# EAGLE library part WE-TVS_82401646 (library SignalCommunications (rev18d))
TVS Diode Super Speed Series Characteristics Operating temperature: –55 ºC to +85 °C for 824 014 x; –40 ºC to +85 °C for 824 016 46 Low clamping voltage Very low capacitance Rail to Rail protection Epoxy flame resistant UL94 V-0 RoHS, REACH and free of halogens Applications Super Speed data lines HDMI 1.3/1.4, DVI DisplayPort USB 3.0 SuperSpeed SATA GBit LAN ESD protection in accordance with EN 61000-4-2 – 8 kV contact discharge – 15 kV air discharge Updated by Dan Xu 2014-07-11 2014 (C) Wurth Elektronik
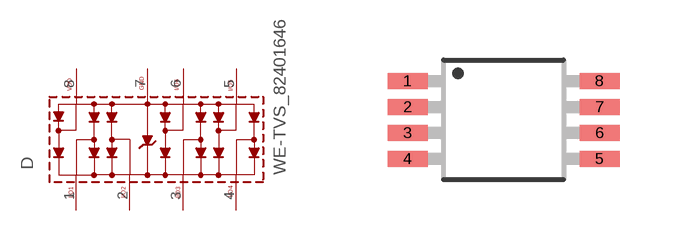
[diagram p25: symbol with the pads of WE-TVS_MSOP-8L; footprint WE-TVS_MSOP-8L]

Designator prefix D

## WE-TVS_82401646  [WE-TVS_MSOP-8L]
1  I/O1
2  I/O2
3  I/O3
4  I/O4  oc
5  I/O5
6  I/O6
7  GND  pwr
8  VDD  pwr

## Footprint WE-TVS_MSOP-8L (pad centres in mm)
TVS Diode Array WE-TVS
smd 1 x 0.4: 1 -2.4,0.975; 2 -2.4,0.325; 3 -2.4,-0.325; 4 -2.4,-0.975; 5 2.4,-0.975; 6 2.4,-0.325; 7 2.4,0.325; 8 2.4,0.975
